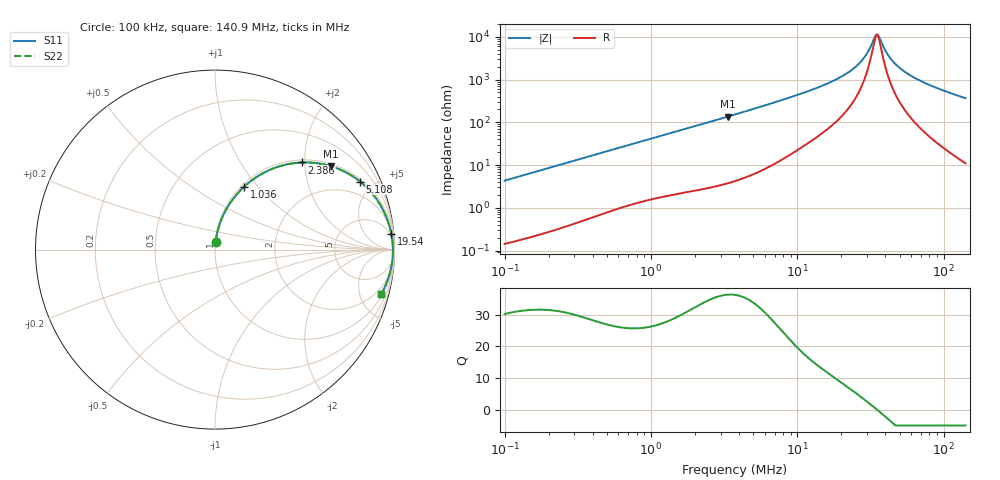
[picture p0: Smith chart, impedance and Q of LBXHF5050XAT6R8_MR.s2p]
! LBXHF5050XAT6R8_MR  S-PARAMETER MODEL  ( General Type )
! Model Generated by TAIYO YUDEN Corporation (http://www.ty-top.com)
! Version 1.0
! TAIYO YUDEN Control No. 201201NI43SB-FBB
! Copyright(c) 2020 TAIYO YUDEN CO.,LTD. All Rights Reserved.
! Product Description (link to TY-COMPAS)
! https://ds.yuden.co.jp/TYCOMPAS/or/detail?pn=LBXHF5050XAT6R8MMR&u=M
! Products Name : Inductors
! Characteristics :
!  Inductance : 6.8 uH , SRF(min) : 25 MHz , DC Resistance(max) : 0.078 Ohm
!  Rated Current : Saturation :3000 mA , Temp Rise : 1350 mA
!  Case Size : 5.0 x 5.0 / 0.197 x 0.197 [mm/inch] , Thickness : 3.1 / 0.122 [mm/inch]
!  (Conditions: Temperature = 25 degC , DC Bias Current/Voltage = 0A / 0V)
! External Node Assignments :
!  1  o---GGG---o  2
! GND o---------o GND
! Frequency Range : 0.1MHz  -  140.89697MHz  [ 402 STEP ]
# MHz S RI R 50
! Freq[MHz].  S11 Real  S11 Imag  S21 Real  S21 Imag  S12 Real  S12 Imag  S22 Real  S22 Imag
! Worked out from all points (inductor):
!   401 points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, 100 kHz to 140.9 MHz, reference 50 ohm
!   read as one part in series: L = 6.84 uH near 103.7 kHz
!   highest Q = 36.3 at 3.367 MHz (marker M1), where L = 6.47 uH
!   self-resonance near 34.89 MHz
!   S11 on the Smith chart (normalised r, x): 100 kHz: 1.00, +0.09; 1.036 MHz: 1.03, +0.85; 2.386 MHz: 1.06, +1.93; 5.108 MHz: 1.13, +4.20; 19.54 MHz: 4, +22; 140.9 MHz: 1.22, -7.34
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0.1  0.00327 0.0429  0.9967 -0.0429  0.9967 -0.0429  0.00327 0.0429
0.336853  0.0245 0.1385  0.9755 -0.1385  0.9755 -0.1385  0.0245 0.1385
0.635287  0.0738 0.2429  0.9262 -0.2429  0.9262 -0.2429  0.0738 0.2429
1.036384  0.1629 0.3508  0.8371 -0.3508  0.8371 -0.3508  0.1629 0.3508
1.134703  0.1869 0.3717  0.8131 -0.3717  0.8131 -0.3717  0.1869 0.3717
2.385857  0.4841 0.4853  0.5159 -0.4853  0.5159 -0.4853  0.4841 0.4853
3.3668  0.648 0.464  0.352 -0.464  0.352 -0.464  0.648 0.464
3.753625  0.6953 0.4467  0.3047 -0.4467  0.3047 -0.4467  0.6953 0.4467
5.108332  0.808 0.3792  0.192 -0.3792  0.192 -0.3792  0.808 0.3792
12.64421  0.9613 0.163  0.0387 -0.163  0.0387 -0.163  0.9613 0.163
19.53556  0.9826 0.0862  0.0174 -0.0862  0.0174 -0.0862  0.9826 0.0862
23.41793  0.9872 0.0582  0.0128 -0.0582  0.0128 -0.0582  0.9872 0.0582
27.07239  0.9896 0.0368  0.0104 -0.0368  0.0104 -0.0368  0.9896 0.0368
29.64065  0.9905 0.0238  0.00949 -0.0238  0.00949 -0.0238  0.9905 0.0238
33.65066  0.9912 0.00577  0.00876 -0.00577  0.00876 -0.00577  0.9912 0.00577
34.89298  0.9913 0.000643  0.00868 -0.000643  0.00868 -0.000643  0.9913 0.000643
36.18117  0.9913 -0.00449  0.00865 0.00449  0.00865 0.00449  0.9913 -0.00449
42.59248  0.9908 -0.0278  0.00924 0.0278  0.00924 0.0278  0.9908 -0.0278
50.13987  0.989 -0.0517  0.011 0.0517  0.011 0.0517  0.989 -0.0517
64.62413  0.9833 -0.0915  0.0167 0.0915  0.0167 0.0915  0.9833 -0.0915
91.19427  0.9675 -0.1535  0.0325 0.1535  0.0325 0.1535  0.9675 -0.1535
140.897  0.9246 -0.2495  0.0754 0.2495  0.0754 0.2495  0.9246 -0.2495
